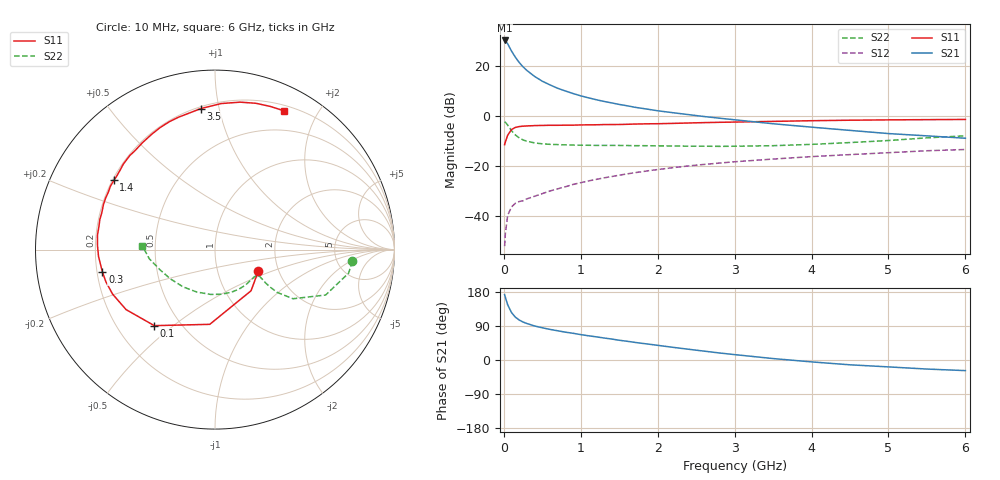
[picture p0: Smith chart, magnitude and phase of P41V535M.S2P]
! SIEMENS Small Signal Semiconductors
! BFP182
! Si NPN RF Bipolar Junction Transistor in SOT143
! VCE = 1.5 V  IC = 35 mA
! Common Emitter S-Parameters:  March  1996
# GHz  S  MA  R  50
!  f  S11  S21  S12  S22
! GHz  MAG  ANG  MAG  ANG  MAG  ANG  MAG  ANG
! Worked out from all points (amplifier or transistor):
!   36 points, 10 MHz to 6 GHz, reference 50 ohm
!   highest |S21| = 30.4 dB at 10 MHz (marker M1)
!   |S21| within 3 dB of that: start of sweep to 78.39 MHz
!   unconditionally stable (mu >= 1): start of sweep to 29.8 MHz; 189.7 MHz to end of sweep
!   at 250 MHz: K = 1.24, MAG = 23.9 dB, |S12| = -33.9 dB
!   at 1.4 GHz: K = 2.05, MAG = 8.9 dB, |S12| = -24.2 dB
!   at 6 GHz: K = 1.49, MAG = -1.9 dB, |S12| = -13.3 dB
!   S11 on the Smith chart (normalised r, x): 10 MHz: 1.57, -0.41; 100 MHz: 0.36, -0.43; 300 MHz: 0.22, -0.09; 1.4 GHz: 0.21, +0.30; 3.5 GHz: 0.21, +0.88; 6 GHz: 0.26, +1.58
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0.01  0.2694 -26.4  32.98 172.5  0.0025 69.4  0.7685 -4.8
0.02  0.3049 -48.8  32.59 165.2  0.0045 73.3  0.7558 -10.0
0.05  0.4174 -94.0  28.19 145.6  0.0104 63.1  0.6665 -22.3
0.1  0.5421 -128.6  20.23 125.0  0.0153 48.7  0.5138 -32.2
0.15  0.5977 -146.0  15.22 113.1  0.0181 44.6  0.4223 -34.5
0.2  0.6221 -156.5  11.93 105.5  0.0196 43.3  0.3685 -34.2
0.25  0.6338 -163.6  9.768 100.1  0.0203 43.2  0.3355 -33.3
0.3  0.6396 -168.7  8.268 96.3  0.0222 44.8  0.3159 -32.3
0.4  0.6502 -176.7  6.274 89.8  0.025 48.7  0.2927 -31.1
0.5  0.6551 178.0  5.034 85.0  0.0282 50.3  0.2803 -31.1
0.6  0.6598 173.0  4.249 80.8  0.0319 53.7  0.274 -31.7
0.7  0.6593 169.1  3.632 77.1  0.0352 55.3  0.2706 -33.0
0.8  0.6631 165.3  3.21 73.5  0.0387 56.3  0.2673 -34.4
1.1  0.6736 154.8  2.339 63.9  0.0507 57.5  0.2624 -40.4
1.4  0.6828 145.6  1.854 55.4  0.0619 57.5  0.2605 -47.3
1.7  0.6981 137.1  1.517 46.6  0.074 55.9  0.2577 -54.9
2.2  0.7199 124.1  1.176 33.4  0.0934 52.2  0.2547 -69.1
2.8  0.7564 109.7  0.916 18.6  0.1153 46.5  0.2495 -88.7
3.5  0.7895 95.8  0.708 3.8  0.139 39.6  0.2574 -113.4
4.5  0.8334 80.3  0.521 -12.7  0.1706 29.7  0.2974 -146.8
5.5  0.8551 68.9  0.405 -23.9  0.2038 19.7  0.3697 -172.1
6  0.8633 63.7  0.363 -28.0  0.2159 14.0  0.4062 176.8
